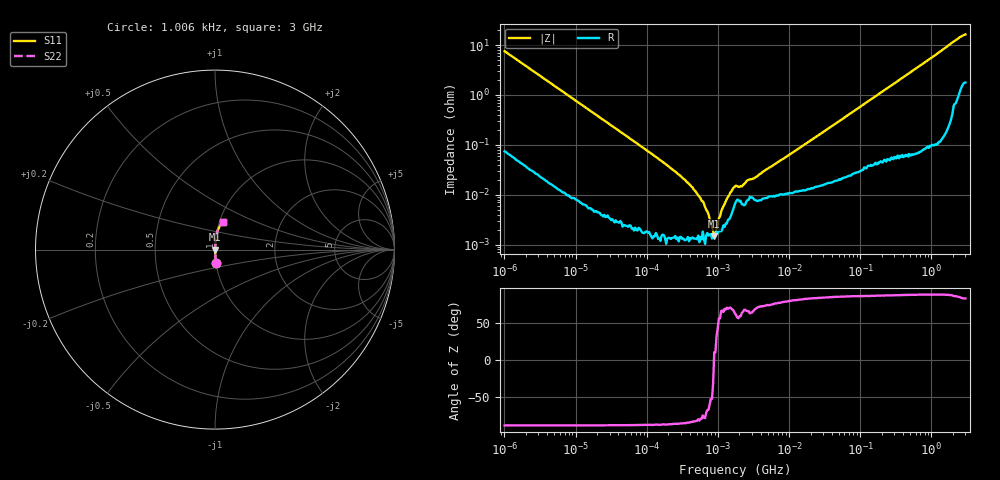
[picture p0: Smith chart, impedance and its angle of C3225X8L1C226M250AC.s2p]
! S-Parameter Data Generated by TDK Corporation
! Copyright(C) 2022 TDK Corporation.
! All Rights Reserved.
! TDK P/N: C3225X8L1C226M250AC (Multilayer Ceramic Chip Capacitor)
! Property: C=22uF
! Size(LxWxT): 3.2x2.5x2.5mm
! Model Type: s2p (Touchstone File Format Version 1.0)
! Frequency: DC=Yes Start=0.001006039MHz Stop=3000MHz 479points Log-sweep
! Model Generated on Apr. 15, 2022
! Port Assignments:
!  1 ---| |--- 2
! Applicable Conditions:
!  Temperature = 25 degC
!  DC Bias Voltage = 0 V
!  Small Signal Operation
! Terms and conditions regarding TDK Simulation Models
! (1)This simulation model is being provided solely for informational purposes. Please refer to the specifications of the products in terms of detailed characteristics of such products.
! (2)In no event shall TDK Corporation of any of its subsidiaries be liable for any loss or damage arising, directly or indirectly,
!  From any information contained in this simulation model, including, but not limited to loss or damages arising from any inaccuracies, omissions or errors in connection with such information.
! (3)Any and all copyrights on this simulation model are owned by TDK Corporation.
!  Duplication or redistribution of this simulation model without prior written permission from TDK Corporation is prohibited.
! (4)This simulation model is subject to any modification or change without any prior notice.
! (5)Neither TDK Corporation nor any of its subsidiaries shall make any warranty, express or implied,
!  Including but not limited to the correctness, implied warranties of merchantability and fitness for a particular purpose with respect to this simulation models.
! (6)The use of this simulation model shall be deemed to have consented to the terms and conditions hereof.
# Hz S MA R 50
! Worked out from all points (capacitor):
!   478 points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, 1.006 kHz to 3 GHz, reference 50 ohm
!   read as one part in series: C = 20.9 uF near 1.083 kHz
!   lowest |Z| = 1.46 mohm at 888.4 kHz (marker M1)
!   series resonance near 881.5 kHz, so ESL is about 1.6 nH
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1006.039  0.07513 -85.1  0.9964 4.3  0.9964 4.3  0.07513 -85.1
2840.326  0.02695 -87.9  0.9994 1.5  0.9994 1.5  0.02695 -87.9
12511.27  0.00618 -89.1  0.9999 0.4  0.9999 0.4  0.00618 -89.1
149930.4  0.0005091 -88.5  1 0.0  1 0.0  0.0005091 -88.5
314670.7  0.0002195 -86.6  1 0.0  1 0.0  0.0002195 -86.6
407891.4  0.0001562 -85.0  1 0.0  1 0.0  0.0001562 -85.0
528728.7  9.765e-05 -81.1  1 0.0  1 0.0  9.765e-05 -81.1
569415.9  8.433e-05 -80.3  1 0.0  1 0.0  8.433e-05 -80.3
888402.1  1.458e-05 10.6  1 -0.0  1 -0.0  1.458e-05 10.6
1386084  9.069e-05 69.7  1 -0.0  1 -0.0  9.069e-05 69.7
1492747  0.0001101 71.5  1 -0.0  1 -0.0  0.0001101 71.5
1668327  0.0001387 66.8  0.9999 -0.0  0.9999 -0.0  0.0001387 66.8
1796709  0.0001519 61.5  0.9999 -0.0  0.9999 -0.0  0.0001519 61.5
2083873  0.0001483 59.5  0.9999 -0.0  0.9999 -0.0  0.0001483 59.5
2701217  0.0001982 66.5  0.9999 -0.0  0.9999 -0.0  0.0001982 66.5
3374034  0.0002227 69.6  0.9999 -0.0  0.9999 -0.0  0.0002227 69.6
4538749  0.0003044 73.9  0.9999 -0.0  0.9999 -0.0  0.0003044 73.9
2.153109e7  0.001306 84.1  0.9999 -0.1  0.9999 -0.1  0.001306 84.1
2.507343e8  0.01423 87.2  0.9994 -0.8  0.9994 -0.8  0.01423 87.2
1.017911e9  0.05653 85.8  0.9974 -3.2  0.9974 -3.2  0.05653 85.8
2.359433e9  0.1333 78.6  0.9823 -7.6  0.9823 -7.6  0.1333 78.6
3e9  0.1584 74.7  0.9703 -9.1  0.9703 -9.1  0.1584 74.7
